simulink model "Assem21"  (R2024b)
settings: Solver=VariableStepAuto  StartTime=0.0  StopTime=5.0  RelTol=1e-3
model workspace: external: MATLAB File (data not in the file)
undefined symbols (not defined in the file or in its folder): deg, kg, Levenberg, m, Marquardt, mm, N, s, smiData, X, Y, Z
libraries: sm_lib x57, nesl_utility x7, robotcorelib x3, robotmaniplib x2
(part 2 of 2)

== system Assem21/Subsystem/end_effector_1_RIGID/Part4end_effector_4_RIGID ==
  ReferenceFrame : sm_lib/Frames and Transforms/Reference Frame
  Solid : sm_lib/Body Elements/File Solid  ExtGeomFileName=Part4-end effector_Default_sldprt.STEP  UnitType=FromFile  ExtGeomFileUnits=m  StepReaderType=HEX  ExportConvexHullGeometry=off  InertiaType=Custom  BasedOnType=DensityFromFile  Density=1000  DensityUnits=kg/m^3  Mass=smiData.Solid(7).mass  MassUnits=kg  CenterOfMass=smiData.Solid(7).CoM  CenterOfMassUnits=mm  MomentsOfInertia=smiData.Solid(7).MoI  MomentsOfInertiaUnits=kg*mm^2  ProductsOfInertia=smiData.Solid(7).PoI  ProductsOfInertiaUnits=kg*mm^2  GraphicType=FromGeometry  MarkerShape=Sphere  MarkerSize=10  GraphicVisPropType=SimpleVisualProperties  GraphicDiffuseColor=smiData.Solid(7).color  GraphicOpacity=smiData.Solid(7).opacity  GraphicSpecularColor=[0.5 0.5 0.5 1.0]  GraphicAmbientColor=[0.15 0.15 0.15 1.0]  GraphicEmissiveColor=[0.0 0.0 0.0 1.0]  GraphicShininess=75  DoExposeReferenceFrame=on  SerializedFrames=<Frames/>
  F : PMIOPort  Side=Left
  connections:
  Solid/RConn1 -- ReferenceFrame/RConn1 -- F/RConn1
